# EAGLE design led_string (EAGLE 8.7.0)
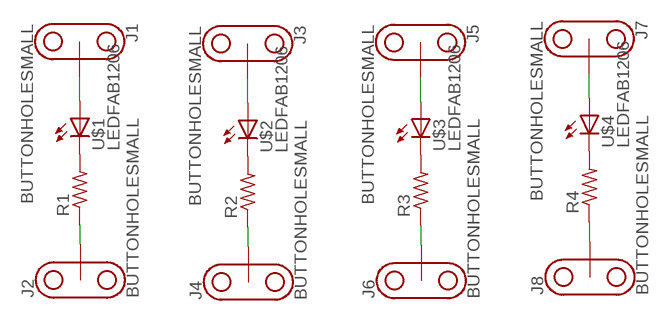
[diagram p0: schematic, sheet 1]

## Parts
J1  BUTTONHOLESMALL  [BUTTONHOLE-SM]
J2  BUTTONHOLESMALL  [BUTTONHOLE-SM]
J3  BUTTONHOLESMALL  [BUTTONHOLE-SM]
J4  BUTTONHOLESMALL  [BUTTONHOLE-SM]
J5  BUTTONHOLESMALL  [BUTTONHOLE-SM]
J6  BUTTONHOLESMALL  [BUTTONHOLE-SM]
J7  BUTTONHOLESMALL  [BUTTONHOLE-SM]
J8  BUTTONHOLESMALL  [BUTTONHOLE-SM]
R1  RES-US1206FAB  [R1206FAB]
R2  RES-US1206FAB  [R1206FAB]
R3  RES-US1206FAB  [R1206FAB]
R4  RES-US1206FAB  [R1206FAB]
U$1  LEDFAB1206  [LED1206FAB]
U$2  LEDFAB1206  [LED1206FAB]
U$3  LEDFAB1206  [LED1206FAB]
U$4  LEDFAB1206  [LED1206FAB]

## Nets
N$1: R1.2 U$1.2(C)
N$2: R2.2 U$2.2(C)
N$3: J3.P$3 U$2.1(A)
N$4: J4.P$3 R2.1
N$5: R3.2 U$3.2(C)
N$6: J5.P$3 U$3.1(A)
N$7: J6.P$3 R3.1
N$8: R4.2 U$4.2(C)
N$9: J1.P$3 U$1.1(A)
N$10: J2.P$3 R1.1
N$11: J7.P$3 U$4.1(A)
N$12: J8.P$3 R4.1

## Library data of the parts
J1-J8 = LilyPad-Wearables:BUTTONHOLE: SparkFun Button Hole - Sewable button holes for connectors
R1-R4 = fab:RES-US: Resistor (US Symbol)
U$1-U$4 = fab:LED: LED

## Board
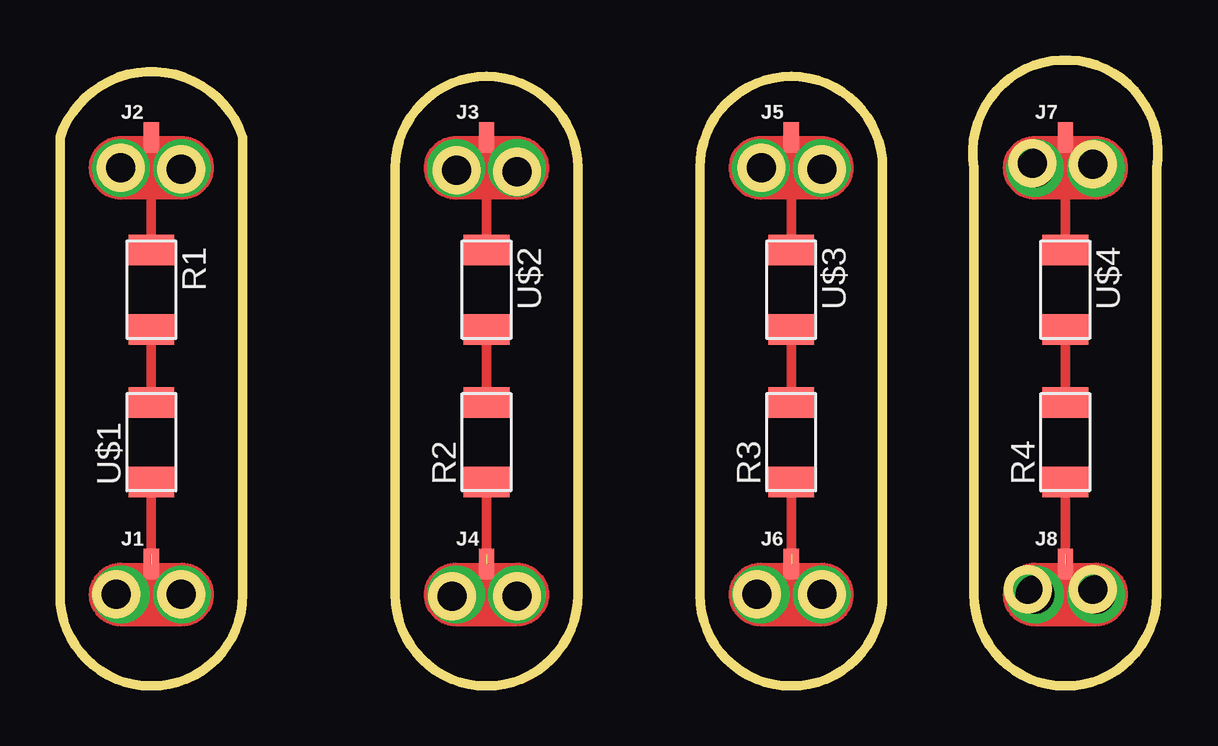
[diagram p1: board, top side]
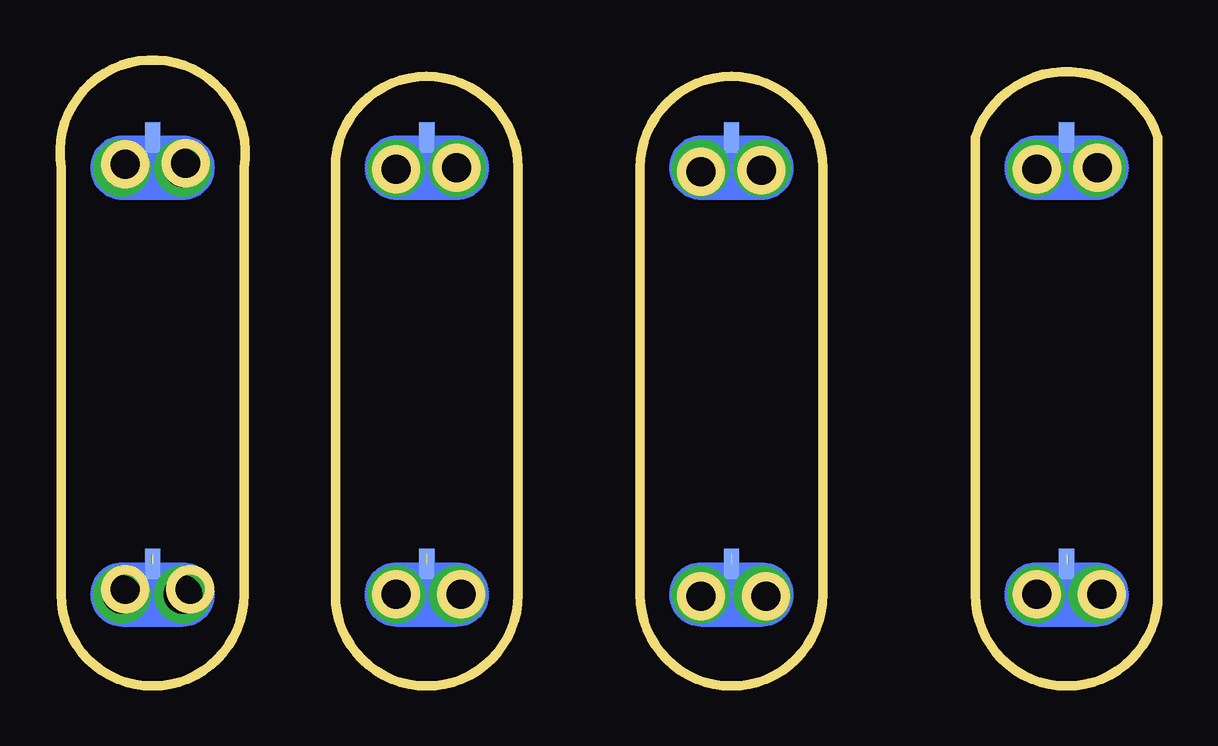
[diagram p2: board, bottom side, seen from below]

Size 45.77 x 26.08 mm. Coordinates in mm from the lower left corner, seen from the top.
Outline: 7.62,22.86 arc143 0,22.86 0,3.81 arc180 7.62,3.81 7.62,22.86
Outline: 21.59,21.59 21.59,3.81 arc-180 13.97,3.81 13.97,21.59 arc-180 21.59,21.59
Outline: 34.29,21.59 34.29,3.81 arc-180 26.67,3.81 26.67,21.59 arc-180 34.29,21.59
Outline: 45.72,21.59 45.72,3.81 arc-180 38.1,3.81 38.1,21.59 arc-199 45.72,21.59
Outline: circle at 2.54,21.59 radius 0.8
Outline: circle at 5.05,21.53 radius 0.8
Outline: circle at 2.35,3.83 radius 0.8
Outline: circle at 5.05,3.83 radius 0.8
Outline: circle at 16.54,21.49 radius 0.8
Outline: circle at 19.05,21.43 radius 0.8
Outline: circle at 16.35,3.73 radius 0.8
Outline: circle at 19.05,3.73 radius 0.8
Outline: circle at 29.24,21.59 radius 0.8
Outline: circle at 31.75,21.53 radius 0.8
Outline: circle at 29.05,3.83 radius 0.8
Outline: circle at 31.75,3.83 radius 0.8
Outline: circle at 40.54,21.79 radius 0.8
Outline: circle at 43.05,21.73 radius 0.8
Outline: circle at 40.35,4.03 radius 0.8
Outline: circle at 43.05,4.03 radius 0.8
Copper layers (1*16): Top 0.035mm / dielectric 1.5mm / Bottom 0.035mm
Design rules "default": minimum track width 6mil, minimum drill 0.35mm, track to track 6mil, track to pad 6mil, pad to pad 6mil, via to via 6mil, smd to smd 6mil, copper to edge 40mil, drill to drill 6mil, minimum pad ring 10mil, minimum via ring 8mil, stop-mask expansion 4mil, vias tented up to drill 0mil, thermal gap 10mil

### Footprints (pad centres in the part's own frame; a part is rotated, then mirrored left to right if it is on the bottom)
BUTTONHOLE-SM = drill 1.6: P$1 -1.27,0; P$2 1.27,0 | smd 0.635 x 1.27: P$3 0,1.27 | smd 0.635 x 1.27 bottom: P$4 0,1.27
R1206FAB = smd 1.27 x 1.905: 1 -1.651,0; 2 1.651,0
LED1206FAB = smd 1.27 x 1.905: 1 -1.651,0; 2 1.651,0

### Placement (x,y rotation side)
J1  3.81,3.81 0 top
J2  3.81,21.59 0 top
J3  17.78,21.59 0 top
J4  17.78,3.81 0 top
J5  30.48,21.59 0 top
J6  30.48,3.81 0 top
J7  41.91,21.59 0 top
J8  41.91,3.81 0 top
R1  3.81,16.51 270 top
R2  17.78,10.16 90 top
R3  30.48,10.16 90 top
R4  41.91,10.16 90 top
U$1  3.81,10.16 90 top
U$2  17.78,16.51 270 top
U$3  30.48,16.51 270 top
U$4  41.91,16.51 270 top

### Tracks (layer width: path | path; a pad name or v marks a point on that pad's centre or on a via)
N$1
  Top 0.4: R1.2 U$1.2
N$2
  Top 0.4: U$2.2 R2.2
N$3
  Top 0.4: J3.P$3 U$2.1
N$4  (1 unrouted)
  Top 0.4: R2.1 17.78,5.5
N$5
  Top 0.4: U$3.2 R3.2
N$6
  Top 0.4: J5.P$3 U$3.1
N$7  (1 unrouted)
  Top 0.4: R3.1 30.48,5.5
N$8
  Top 0.4: U$4.2 R4.2
N$9  (1 unrouted)
  Top 0.4: U$1.1 3.81,5.5
N$10
  Top 0.4: J2.P$3 R1.1
N$11
  Top 0.4: J7.P$3 U$4.1
N$12  (1 unrouted)
  Top 0.4: R4.1 41.91,5.5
